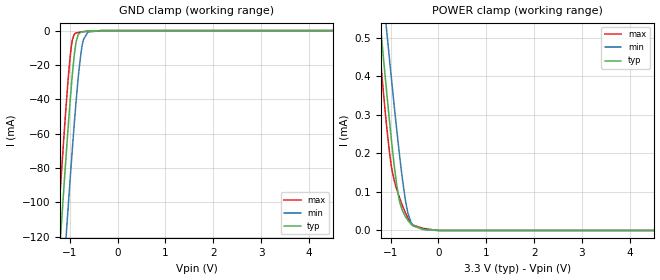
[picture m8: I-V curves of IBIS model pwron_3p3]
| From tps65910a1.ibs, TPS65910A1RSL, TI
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|   pwron_3p3 Model
[Model]   pwron_3p3
Model_type   Input
Vinl = 0.99
Vinh = 2.31
|   typ   min   max
|   (nom PVT)   (fast PVT)   (slow PVT)
C_comp   1.631e-13   1.628e-13   1.641e-13
[Model spec]
|subparameter
Vinl   0.99   0.945   1.035
Vinh   2.31   2.205   2.415
| Where nom  PVT is Nominal Process, 3.3V, 27C
|   Fast PVT is Strong Process,  3.45V, -40C
|   Slow PVT is Weak Process,   3.15V, 125C
[Voltage Range]   3.3   3.15   3.45
|Junction Temperature
[Temperature Range]   27   125   -40
[Power Clamp Reference]   3.3   3.15   3.45
[GND Clamp Reference]   0   0   0
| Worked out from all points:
|   GND clamp passes 1 mA (typ) near -0.76 V on its own axis
[GND Clamp]
|   Voltage   I(typ)   I(min)   I(max)
-3.3V     -1.066A    -1.108A    -1.042A
-1.251V   -145mA     -192.9mA   -115.3mA
-1.227V   -134.8mA   -182.7mA   -105mA
-1.127V   -93.2mA    -140.9mA   -63.63mA
-1.07V    -70.49mA   -117.7mA   -41.57mA
-966.9mV  -32.56mA   -77.15mA   -9.33mA
-940.2mV  -24.04mA   -67.11mA   -4.865mA
-871.3mV  -7.489mA   -42.72mA   -1.465mA
-809.1mV  -1.863mA   -23.65mA   -1.037mA
-735.9mV  -756.6uA   -7.991mA   -725.4uA
-622.5mV  -354uA     -856.5uA   -328.8uA
6.6V      0A         0A         0A
[POWER Clamp]
|   Voltage   I(typ)   I(min)   I(max)
-3.3V     3.547mA    3.55mA     3.698mA
-1.282V   626.5uA    775.8uA    544.3uA
-1.196V   509.1uA    663.5uA    420.8uA
-1.082V   359.4uA    518.6uA    269.7uA
-967.8mV  217.4uA    375.7uA    154.7uA
-867.9mV  114.3uA    256.8uA    105.5uA
-821.7mV  80.99uA    204.8uA    88.2uA
-684.9mV  35.14uA    74.56uA    44.54uA
-640.2mV  26.57uA    46.15uA    33.17uA
-531.2mV  11.63uA    13.41uA    14.03uA
1.2mV     0A         0A         0A
6.6V      0A         0A         0A
